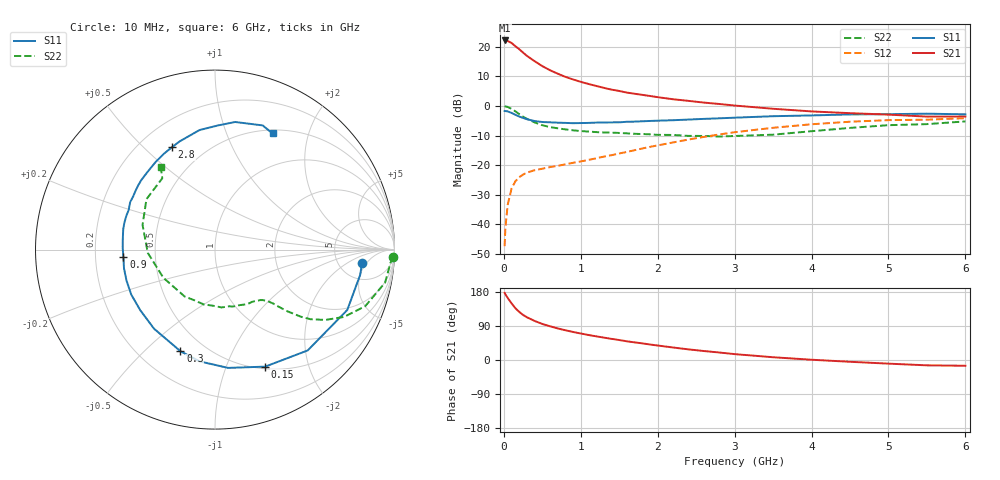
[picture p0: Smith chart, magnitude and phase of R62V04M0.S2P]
! SIEMENS Small Signal Semiconductors
! BFR193
! Si NPN RF Bipolar Junction Transistor in SOT23
! VCE = 2 V  IC = 4 mA
! Common Emitter S-Parameters:  May  1996
# GHz  S  MA  R  50
!  f  S11  S21  S12  S22
! GHz  MAG  ANG  MAG  ANG  MAG  ANG  MAG  ANG
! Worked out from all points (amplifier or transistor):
!   36 points, 10 MHz to 6 GHz, reference 50 ohm
!   highest |S21| = 22.1 dB at 10 MHz (marker M1)
!   |S21| within 3 dB of that: start of sweep to 202.6 MHz
!   unconditionally stable (mu >= 1): 947.1 MHz to 2.022 GHz
!   at 250 MHz: K = 0.37, MSG = 20.6 dB, |S12| = -23.2 dB
!   at 1.4 GHz: K = 1.09, MAG = 9.3 dB, |S12| = -16.6 dB
!   at 6 GHz: K = 0.98, MSG = 0.3 dB, |S12| = -4.1 dB
!   S11 on the Smith chart (normalised r, x): 10 MHz: 8.47, -3.92; 150 MHz: 0.53, -1.38; 300 MHz: 0.37, -0.65; 900 MHz: 0.32, -0.03; 2.8 GHz: 0.33, +0.61; 6 GHz: 0.54, +1.47
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0.01  0.8231 -5.2  12.76 177.0  0.0043 88.0  0.9941 -2.3
0.02  0.8208 -9.9  12.52 173.4  0.0087 85.3  0.9802 -4.4
0.05  0.8102 -24.5  12.49 163.9  0.0214 77.6  0.9653 -11.0
0.1  0.7631 -47.4  11.58 149.5  0.0402 67.5  0.8947 -20.6
0.15  0.7094 -66.8  10.19 136.8  0.0537 58.6  0.8117 -27.5
0.2  0.6631 -83.7  9.095 126.9  0.0628 52.9  0.7293 -32.5
0.25  0.6284 -98.0  7.953 118.9  0.0694 48.6  0.6582 -36.1
0.3  0.5978 -108.8  7.013 112.8  0.0751 46.5  0.6076 -38.0
0.4  0.5565 -127.6  5.7 103.1  0.0823 43.5  0.5282 -40.5
0.5  0.5363 -140.9  4.707 95.1  0.0873 43.0  0.4732 -42.0
0.6  0.5296 -151.8  4.011 89.0  0.093 43.9  0.4402 -42.9
0.7  0.5224 -160.7  3.508 83.4  0.0976 44.9  0.4196 -43.9
0.9  0.5122 -175.6  2.804 74.0  0.1099 48.1  0.3878 -46.5
1.1  0.5177 172.7  2.353 66.0  0.1229 51.9  0.3696 -50.5
1.3  0.5267 163.5  2.021 59.1  0.1396 54.5  0.3568 -54.7
1.6  0.5415 150.8  1.681 49.3  0.1677 57.2  0.3451 -62.9
2.2  0.5746 130.3  1.298 33.0  0.2423 57.1  0.3243 -83.6
2.8  0.619 112.8  1.08 19.8  0.3301 51.2  0.305 -112.1
3.5  0.6716 97.4  0.897 7.3  0.4285 40.1  0.3277 -151.4
4.5  0.7198 81.0  0.756 -4.7  0.5422 22.5  0.4263 161.2
5.5  0.7411 69.0  0.661 -14.1  0.5865 5.1  0.4939 126.5
6  0.7222 63.6  0.664 -15.2  0.6223 0.0  0.5489 123.3
